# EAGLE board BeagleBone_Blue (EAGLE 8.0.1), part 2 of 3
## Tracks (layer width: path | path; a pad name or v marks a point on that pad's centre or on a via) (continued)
GND  (via drill 0.25 pad 0.46, 0.41, 0.5) (continued)
  Top 0.406: H2.3 79.3,24.38 | H2.4 79.96,24.41 | 83.84,22.52 83.84,24.43 | H2.9 83.21,24.43 | H2.18 81.92,27.46 | H1.9 74.65,16.76 | H1.10 74.65,17.41 74.65,17.4 | H1.3 74.62,12.86 74.62,12.85 | H1.4 74.62,13.51 | 74.62,13.51 | C38.2 46.13,45.99 v46.13,44.83 | C3.2 v49.15,42.88 | D9.A v60.45,53.39 | H1.18 71.6,15.46 71.6,15.47 | 5VREG.4 52.32,46.6 52.58,46.86 v52.58,47.62 | C5.2 50.64,43.3 v50.22,42.88 | R64.1 R63.1 R62.1 R61.1 R21.2 R22.2 20.75,2.23 v20.5,2.49
  Bottom 0.152: U13.H10 30.62,34.44 v31.62,34.44 | v31.62,34.44 32.62,34.44 U13.G5 33.12,34.69 v33.38,34.95 v33.37,34.95 U13.C4 | U13.K8 31.62,33.44 v31.62,34.44 | U13.E7 31.62,35.44 v31.62,34.44 | U13.N5 U13.P6 32.36,31.19 32.72,30.84 33.02,30.84 U13.P4 33.73,30.84 34.04,30.84 34.37,31.17 U13.N2 34.37,31.21 34.39,31.19 34.39,31.17 34.72,30.84 35.03,30.84 35.89,31.7 v35.89,32.51 | X2.6 3.36,31.03 v3.38,31.01 | X2.GND 15.76,28.79 15.93,28.96 v16.84,28.96 | 56.03,40.66 R143.1 56.03,40.56 56.16,40.44 v56.57,40.44 | R16.1 v65.15,37.85 | R17.1 v65.15,36.7 | R129.1 64.95,35.56 65.15,35.76 v65.15,36.04 | R135.1 v65.15,34.42 | R115.1 v65.15,30.99 | R131.1 v65.15,32.13 | R113.1 v65.18,29.84 | R25.2 v69.22,10.92 | R110.2 56.39,14.45 56.54,14.6 v56.97,14.6 | R14.2 58.73,14.45 58.88,14.6 v59.31,14.6 | v58.22,20.37 58.22,19.91 58.4,19.74 R158.2 | C27.2 v32.21,6.93 | C40.2 v48.9,9.55 | R59.1 49.35,10.77 49.25,10.87 49.25,11.02 49.15,11.12 v48.69,11.12 | v60.27,17.53 60.27,18.41 C41.2
  Bottom 0.254: C23.1 v67.74,22.02 | TP12.TP v69.39,2.64 | C2.1 v76.2,19.89 | C25.2 v29.59,52.83 | C26.2 v31.11,52.83 | C20.1 52.06,52.44 52.32,52.7 52.32,53.01 v52.7,53.39 | R48.1 C21.1 53.8,51 R46.1 53.77,51.49 53.85,51.56 53.85,53.37 v53.87,53.39 | U4.4 5.53,9.52 C55.2 6.15,9.58 v6.48,9.91 | C34.1 v14.43,16.38 | v19.33,37.72 19.33,39.29 C52.2 | U9.TP 21.84,38.25 22.43,38.84 23.55,38.84 v24.13,38.25 | U9.11 22.6,37.8 22.91,37.8 23.19,38.08 v23.19,38.23 | R108.2 R89.2 22.84,27.18 v21.77,26.11 | C51.1 22.81,30.73 v23.24,31.17 | C49.1 v41.66,38.86 | C16.2 v49.81,8.2 | R150.2 v36.8,32.51 | R24.2 13.97,43.94 13.44,44.48 v11.58,44.48 | R47.1 55.24,46.53 55.4,46.38 55.4,46.05 55.5,45.95 v55.5,45.49 | C24.1 55.96,47.62 56.87,48.54 v58.22,48.54 | U5.2 v21.18,19.63 | C62.2 v17.63,7.14 | C28.2 v21.01,18.41 | C45.2 v16.28,9.45 | C61.1 20.45,14.07 v20.75,14.38 | C63.2 v24.69,12.09 | C33.2 22.89,14.63 v23.67,14.63 | U1.2 v36.2,11.05 | C46.2 17.87,15.08 18.16,15.37 v18.54,15.37
  Bottom 0.406: L4.1 v15.11,6.86 | X4.GND 5.13,39.65 5.38,39.9 5.38,43 v3.58,44.81 | D1.A 51.42,43.31 50.65,43.31 v50.22,42.88
  Bottom 0.813: R107.1 14.82,44.23 14.1,44.96 14.1,45.95 13.54,46.51 5.23,46.51 4.47,47.27 12V.OUT
  other vias: 6.22,25.78 6.22,27.05 6.22,28.32 6.22,29.59 6.22,30.86 6.22,32.13 6.22,33.4 6.22,34.67 6.22,35.94 7.49,35.94 8.76,35.94 12.57,35.94 11.3,33.4 11.3,34.67 11.3,30.86 10.03,30.86 8.76,30.86 7.49,30.86 7.49,25.78 8.76,25.78 10.03,25.78 11.3,25.78 11.3,27.05 11.3,28.32 11.3,29.59 12.57,30.86 13.84,30.86 16.38,33.4 16.38,32.13 16.38,28.32 16.38,27.05 16.38,25.78 15.11,25.78 13.84,25.78 12.57,25.78 16.38,35.94 15.11,35.94 18.16,51.94 18.16,52.83 19.05,51.94 20.83,52.83 19.05,52.83 19.94,52.83 19.94,51.94 20.83,51.94 37.47,52.96 36.45,52.96 35.43,52.96 34.42,52.96 33.4,52.96 37.47,50.42 36.45,50.42 35.43,50.42 33.4,50.42 34.42,50.42 13.84,35.94 16.38,34.67 10.03,35.94 11.3,35.94 15.11,30.86 16.38,30.86 16.38,29.59 4.06,26.67 3.17,26.67 2.29,26.67 5.08,23.88 5.08,22.99 5.08,22.1 4.32,20.83 3.56,20.83 4.32,20.07 3.56,20.07 2.79,22.1 2.79,22.99 2.79,23.88 2.79,24.77 2.79,25.65 6.58,42.04 6.58,41.22 6.48,40.41 6.1,39.57 6.58,42.85 40.36,23.75 40.36,40.56 41.63,40.56 42.95,40.56 50.6,40.67 51.77,40.67 61.65,40.39 62.33,40.39 50.5,26.42 51.79,25.17 53.09,27.48 54.33,26.42 53.06,26.44 51.79,26.42 51.82,27.51 50.52,27.69 48.13,30.38 50.52,28.57 54.33,25.15 49.28,29.16 53.06,25.15 49.23,40.67 48.01,40.67 40.34,22.68 54.36,32.51 55.63,26.11 54.36,27.38 50.55,25.17 20.7,5.21 20.7,5.97
  pour Route15 (rank 6): -1.27,55.88 87.63,55.88 87.63,-1.27 -1.27,-1.27
  pour Top (no thermals): 21.21,49.66 21.21,52.96 26.42,52.96 26.42,49.91 31.5,49.91 31.5,53.47 17.53,53.47 17.53,50.29 19.94,50.29 19.94,49.66
  pour Bottom (no thermals): 38.23,53.47 32.77,53.47 32.77,49.91 38.23,49.91
  pour Top (no thermals): 38.61,53.47 32,53.47 32,49.91 38.61,49.91
  pour Top (rank 4): 1.52,43.69 21.21,43.69 21.21,20.19 16.26,20.19 16.26,17.91 1.52,17.91
  pour Top: 75.18,10.8 75.18,21.84 77.22,21.84 77.22,24 84.84,24 84.84,27.81 76.2,27.81 76.2,29.59 73.66,29.59 73.66,25.27 73.03,25.27 73.03,20.32 71.12,20.32 71.12,10.8
  pour Bottom: 17.78,53.34 21.21,53.34 21.21,51.56 17.78,51.56
  pour Top (rank 3): 39.75,20.7 39.75,41.02 62.61,41.02 62.61,39.75 42.29,39.75 42.29,37.21 41.02,37.21 41.02,20.7
  pour Top: 47.37,32.13 47.37,30.86 49.91,28.32 49.91,24.51 52.45,24.51 53.72,23.24 54.99,23.24 54.99,24.51 56.26,25.78 57.53,25.78 57.53,30.86 54.99,33.4 53.72,33.4 52.45,32.13 51.18,32.13 49.91,30.86 48.64,32.13
  pour Bottom (rank 3, no thermals): 20.45,9.52 20.45,4.83 20.95,4.83 20.95,9.52
GNDA_ADC  (via drill 0.25 pad 0.46)
  Top 0.152: 53.8,16.89 SIP.A9 53.72,17.32 54.23,17.83 54.23,18.09 54.81,18.67 54.81,18.92 54.51,19.23 54.51,19.69 54.69,19.86 54.69,20.32 54.51,20.5 54.51,21.03 v54.81,21.34 54.99,21.51 SIP.E8 | SIP.A6 57.53,16.59 v57.23,16.28
  Bottom 0.152: v57.23,16.28 56.52,16.99 56.52,17.93 56.67,18.09 56.87,18.09 57.07,18.29 C42.2 C43.2 C44.2 57.07,21.34 56.92,21.49 54.97,21.49 v54.81,21.34
GPIO1_17  (via drill 0.25 pad 0.46)
  Top 0.152: GP0.4 45.18,6.59 45.62,6.15 v45.97,6.15 | SIP.V14 48.16,37.69 48.16,37.01 48.36,36.8 v48.36,36.58 | v65.46,16.92 64.95,16.41 63.68,16.41 63.4,16.69 63.4,17.14 62.99,17.55 v62.26,17.55
  Bottom 0.152: v65.46,16.92 65.46,20.37 64.75,21.08 64.75,22.5 55.88,31.37 53.16,31.37 51.46,33.07 51.46,33.63 51.13,33.96 50.09,33.96 49.45,34.59 49.45,35.48 v48.36,36.58 | v62.26,17.55 62.48,17.32 62.48,6.68 61.77,5.97 46.15,5.97 v45.97,6.15
GPIO1_25  (via drill 0.25 pad 0.46)
  Top 0.152: GP0.3 46.23,8.84 46.23,7.95 46.56,7.62 v46.56,6.48 | SIP.U16 44.83,36.8 v45.06,36.58
  Bottom 0.152: v46.56,6.48 46.76,6.27 61.65,6.27 62.18,6.81 62.18,16.18 61.77,16.59 61.77,21.54 54.71,28.6 52.05,28.6 49.78,30.86 49.53,30.86 48.23,32.16 48.23,32.36 47.57,33.02 47.3,33.02 46.66,33.66 46.66,34.39 46.23,34.82 46.23,35.51 45.64,36.09 45.36,36.09 45.06,36.4 v45.06,36.58
GPIO3_1  (via drill 0.25 pad 0.46)
  Top 0.152: SIP.H17 43.56,25.25 43.81,24.99 46.3,24.99 46.74,24.56 v46.74,24.21 | GP1.4 v35.03,6.15 | v35.15,18.49 35.15,17.35 34.24,16.43 33.53,16.43 v33.35,16.61
  Bottom 0.152: v46.74,24.21 46.74,24.03 46.35,23.65 45.09,23.65 44.83,23.39 44.12,23.39 41.71,20.98 40.59,20.98 38.43,18.82 35.48,18.82 v35.15,18.49 | v35.03,6.15 34.85,5.97 31.9,5.97 31.19,6.68 27.13,6.68 26.06,7.75 26.06,15.57 27.28,16.79 33.17,16.79 v33.35,16.61
GPIO3_2  (via drill 0.25 pad 0.46)
  Top 0.152: SIP.J15 46.48,27.05 47.27,26.26 47.57,26.26 47.85,25.98 47.85,24.08 v47.65,23.88 | GP1.3 36.04,4.59 v36.04,6.63 | v35.81,18.34 35.81,17.3 34.65,16.13 32.89,16.13 v32.72,16.31
  Bottom 0.152: v47.65,23.88 47.12,23.34 45.24,23.34 44.98,23.09 44.25,23.09 41.83,20.68 40.72,20.68 38.56,18.52 35.99,18.52 v35.81,18.34 | v36.04,6.63 34.77,6.63 34.42,6.27 32.05,6.27 31.34,6.98 27.25,6.98 26.36,7.87 26.36,15.44 27.41,16.48 32.54,16.48 v32.72,16.31
GPIO3_17  (via drill 0.25 pad 0.46)
  Top 0.152: SIP.C12 v50.55,18.8 | v46.13,11.25 44.15,11.25 43.18,10.29 GP0.6
  Bottom 0.152: v50.55,18.8 49.25,18.8 48.62,18.16 48.62,16.38 46.94,14.71 46.76,14.71 46,13.95 46,12.95 46.61,12.34 46.61,11.73 v46.13,11.25
GPIO3_20
  Top 0.152: GP0.5 44.18,9.91 44.78,10.52 46.13,10.52 46.61,11 46.61,12.14 47.04,12.57 47.65,12.57 48.67,13.59 48.67,14.4 49.43,15.16 49.43,18.14 48.69,18.87 48.41,18.87 48.16,19.13 48.16,19.66 48.64,20.14 SIP.D13
I2C0_SCL  (via drill 0.25 pad 0.46)
  Top 0.152: SIP.C16 44.83,19.1 44.73,19 v44.25,19 | SIP.C20 38.94,18.62 38.94,16.53 38.56,16.15 v38.15,16.15
  Bottom 0.152: R23.1 25.76,20.27 28.02,18.01 35.41,18.01 37.26,16.15 v38.15,16.15 38.41,16.15 41.25,19 v44.25,19
  Bottom 0.254: U5.1 22.99,20.57 23.29,20.27 R23.1
I2C0_SDA  (via drill 0.25 pad 0.46)
  Top 0.152: SIP.C17 43.56,18.8 43.71,18.64 43.89,18.64 v44.2,18.34 | SIP.C19 40.34,18.74 39.55,18.74 39.24,18.44 39.24,16.15 v38.76,15.67
  Bottom 0.152: R2.1 26.59,19 27.89,17.7 35.28,17.7 37.31,15.67 v38.76,15.67 38.76,16.08 41.02,18.34 v44.2,18.34
  Bottom 0.254: U5.3 22.96,18.69 23.27,19 R2.1
I2C1_SCL  (via drill 0.25 pad 0.46)
  Top 0.152: SIP.A16 44.83,16.36 44.96,16.23 v44.96,15.8 | v36.4,7.7 36.05,8.04 I2C.3
  Bottom 0.152: v44.96,15.8 44.78,15.62 40.69,15.62 39.65,14.58 34.04,14.58 32.74,13.28 32.74,9.73 33.71,8.76 35.33,8.76 v36.4,7.7 36.4,7.37 36.6,7.16 R12.1
I2C1_SDA  (via drill 0.25 pad 0.46)
  Top 0.152: v44.35,16.1 44.35,17.09 44.83,17.58 SIP.B16 | v35.71,7.7 35.28,7.7 35.05,7.92 I2C.4
  Bottom 0.152: v44.35,16.1 44.17,15.93 40.56,15.93 39.52,14.88 33.91,14.88 32.44,13.41 32.44,9.6 33.58,8.46 34.31,8.46 35.08,7.7 v35.71,7.7 35.71,7.31 35.56,7.16 R13.2
I2C2_SCL  (via drill 0.25 pad 0.46)
  Top 0.152: BMP.4 28.46,23.1 | BMP.4 28.21,23.05 27.96,23.29 R11.1 27.48,23.67 27.28,23.88 25.45,23.88 25.17,24.16 25.17,24.87 25.3,24.99 26.87,24.99 27.18,25.3 27.18,26.57 27.32,26.7 IMU.23 | BMP.4 28.46,22.72 28.93,22.25 32.69,22.25 33.12,21.82 35.69,21.82 37.19,20.32 v37.19,18.03 | SIP.D17 43.87,21.01 v43.87,21.36
  Bottom 0.152: v43.87,21.36 42.95,21.36 41.96,20.37 40.84,20.37 38.68,18.21 37.36,18.21 v37.19,18.03
I2C2_SDA  (via drill 0.25 pad 0.46)
  Top 0.152: BMP.3 29.11,23.11 | BMP.3 29.11,23.41 28.98,23.55 28.37,23.55 28.22,23.7 28.22,24.13 27.89,24.46 R10.2 27.48,25.83 27.71,26.06 IMU.24 | BMP.3 29.11,22.73 29.29,22.55 32.84,22.55 33.27,22.12 35.84,22.12 37.67,20.3 v37.67,17.58 | SIP.D18 42.29,20.4 v42.6,20.09
  Bottom 0.152: v37.67,17.58 38,17.91 38.81,17.91 40.97,20.07 42.57,20.07 v42.6,20.09
IMU_INT  (via drill 0.25 pad 0.46)
  Top 0.152: 31.16,28.3 IMU.12 31.84,28.3 32.23,27.91 32.23,24.51 32.51,24.23 32.51,23.34 33.43,22.43 35.97,22.43 38.15,20.24 v38.15,17.12 | SIP.A14 47.37,17.22 v46.76,17.83
  Bottom 0.152: v38.15,17.12 38.15,17.37 38.38,17.6 38.94,17.6 40.95,19.61 42.88,19.61 43.38,20.12 44.5,20.12 45.03,19.58 45.03,18.29 45.49,17.83 v46.76,17.83
L3
  Top 0.254: B2.C R33.1
L4
  Top 0.254: B3.C R32.1
LDO_PGOOD
  Top 0.152: SIP.B5 59.28,18.64 59.28,19.69 59.05,19.91 58.42,19.91 58.01,19.51 58.01,19.15 57.81,18.95 57.33,18.95 57.05,19.23 57.05,19.79 56.62,20.22 56.03,20.22 55.47,20.78 55.47,22.17 55.19,22.45 50.95,22.45 50.72,22.23 50.37,22.23 50.14,22.45 41.96,22.45 41.81,22.3 41.81,21.03 41.5,20.73 41.5,19.13 41.1,18.72 40.87,18.72 40.31,18.16 SIP.B20
LED_GRN  (via drill 0.25 pad 0.46)
  Top 0.152: SIP.T7 56.26,35.46 55.78,34.98 55.78,33.2 56.06,32.92 56.67,32.92 57.05,32.54 57.05,31.88 57.33,31.6 57.61,31.6 58.01,31.19 58.01,25.73 58.45,25.3 63.14,25.3 v63.22,25.38 | v24.66,5.46 22.61,5.46 22.35,5.71 G.A 22.35,7.42 22.63,7.7 31.09,7.7 31.73,7.06 31.73,5.03 32.18,4.57 GP1.6
  Bottom 0.152: v63.22,25.38 62.76,25.83 62.76,26.36 62.97,26.57 63.48,26.57 64.01,26.04 64.01,24.54 65.66,22.88 65.66,21.49 66.67,20.47 66.67,15.95 64.31,13.59 64.31,5.92 62.53,4.14 25.2,4.14 24.66,4.67 v24.66,5.46
LED_RED  (via drill 0.25 pad 0.46)
  Top 0.152: 56.26,34.7 SIP.R7 56.26,34.14 57.05,33.35 57.05,33.12 57.25,32.92 57.58,32.92 58.01,32.49 58.01,31.7 58.32,31.39 58.32,26.7 58.75,26.26 63.07,26.26 v63.25,26.09 | R.A 23.88,7.01 24.08,7.21 v24.64,7.21 27.76,7.21 27.94,7.39 30.96,7.39 31.42,6.93 31.42,4.14 32.03,3.53 33.81,3.53 34.02,3.74 GP1.5
  Bottom 0.152: v63.25,26.09 63.7,25.63 63.7,24.41 65.35,22.76 65.35,21.36 66.37,20.34 66.37,16.08 64.01,13.72 64.01,6.05 62.41,4.45 25.63,4.45 25.4,4.67 25.4,6.83 25.02,7.21 v24.64,7.21
MCASP0_ACLKR  (via drill 0.25 pad 0.46)
  Top 0.152: SIP.U18 41.66,36.58 v41.66,36.12 | 23.99,31.89 U10.20 23.99,31.99 24.18,32.18 25.32,32.18 25.93,32.79 26.95,32.79 27.36,33.2 27.36,34.04 27.51,34.19 v27.84,34.19
  Bottom 0.152: v41.66,36.12 41.17,36.12 40.28,35.23 40.28,32.08 39.5,31.29 35.92,31.29 35.15,30.53 32.54,30.53 28.88,34.19 v27.84,34.19
MCASP0_AXR0  (via drill 0.25 pad 0.46)
  Top 0.152: SIP.T16 44.07,35.18 v44.07,34.24 | U10.17 25.57,29.98 25.93,30.35 25.93,31.93 26.19,32.18 v27.84,32.18
  Bottom 0.152: v44.07,34.24 43.54,34.77 41.45,34.77 41.2,34.52 41.2,31.7 39.88,30.38 36.3,30.38 35.53,29.62 31.95,29.62 29.38,32.18 v27.84,32.18
MCASP0_AXR1  (via drill 0.25 pad 0.46)
  Top 0.152: SIP.V17 43.08,38 43.08,35.43 v43.26,35.25 | v27.84,33.5 28.19,33.5 28.32,33.38 28.32,31.88 28.14,31.7 27.58,31.7 27.41,31.88 26.39,31.88 26.24,31.72 26.24,30 25.73,29.49 U10.16
  Bottom 0.152: v43.26,35.25 42.72,35.79 42.22,35.79 41.96,35.53 41.02,35.53 40.59,35.1 40.59,31.95 39.62,30.99 36.04,30.99 35.28,30.23 32.34,30.23 28.89,33.68 28.02,33.68 v27.84,33.5
MCASP0_FSR  (via drill 0.25 pad 0.46)
  Top 0.152: SIP.V12 49.43,38.96 43.08,38.96 42.77,38.66 42.77,35.41 42.67,35.31 v42.47,35.31 | U10.18 25.51,30.48 25.63,30.61 25.63,32.05 26.06,32.49 27.1,32.49 27.46,32.84 v27.84,32.84
  Bottom 0.152: v42.47,35.31 42.39,35.23 41.15,35.23 40.89,34.98 40.89,31.83 39.75,30.68 36.17,30.68 35.41,29.92 32.14,29.92 29.38,32.69 27.99,32.69 v27.84,32.84
MDIR_1A  (via drill 0.25 pad 0.46)
  Top 0.152: H1.21 68.25,13.51 67.46,14.3 67.46,16.03 66.98,16.51 66.98,17.65 66.52,18.11 v64.67,18.11 | SIP.T13 49.4,35.18 49.4,34.47 49.68,34.19 50.14,34.19 50.55,33.78 v50.55,33.17
  Bottom 0.152: v64.67,18.11 64.85,18.29 64.85,20.07 64.14,20.78 64.14,22.23 55.6,30.76 52.91,30.76 50.55,33.12 v50.55,33.17
MDIR_1B  (via drill 0.25 pad 0.46)
  Top 0.152: H1.22 68.19,12.86 v67.79,13.26 | v61.7,15.98 62,15.98 62.36,15.62 64.59,15.62 v66.37,13.84 | SIP.U17 44.12,37.21 44.4,36.93 v44.4,36.55
  Bottom 0.152: v67.79,13.26 67.21,13.84 v66.37,13.84 | v61.7,15.98 61.47,16.2 61.47,21.41 54.59,28.3 51.92,28.3 49.66,30.56 49.4,30.56 47.93,32.03 47.93,32.23 47.45,32.72 47.17,32.72 46.35,33.53 46.35,34.27 45.92,34.7 45.92,35.38 45.52,35.79 45.03,35.79 44.4,36.42 v44.4,36.55
MDIR_2A  (via drill 0.25 pad 0.46)
  Top 0.152: H1.17 67.81,16.11 67.28,16.64 67.28,17.91 66.4,18.8 v62.87,18.8 | SIP.R13 48.08,34.11 v47.75,34.11
  Bottom 0.152: v62.87,18.8 62.87,21.74 55.09,29.52 52.43,29.52 50.16,31.77 49.91,31.77 49.15,32.54 49.15,32.74 47.78,34.11 v47.75,34.11
MDIR_2B  (via drill 0.25 pad 0.46)
  Top 0.152: SIP.V4 60.07,38.02 60.76,37.34 v60.76,36.73 | v67.89,16.76 H1.16 | v65.43,27.03 64.62,27.84 60.81,27.84 60.55,28.09 60.55,31.11 60.91,31.47 v62.33,31.47
  Bottom 0.152: v67.89,16.76 67.59,17.07 67.59,20.88 66.57,21.89 66.57,24.21 65.73,25.04 65.73,26.72 v65.43,27.03 | v60.76,36.73 61.06,36.42 61.32,36.42 61.49,36.25 61.49,35.92 61.77,35.64 62,35.64 62.41,35.23 62.41,34.75 62.66,34.49 62.66,34.14 62.97,33.83 63.17,33.83 63.32,33.68 R140.1 62.84,33.27 62.33,32.77 v62.33,31.47
MDIR_3A  (via drill 0.25 pad 0.46)
  Top 0.152: SIP.R4 60.53,34.67 v61.16,34.04 | H2.21 79.93,29.86 v79.93,30.94
  Bottom 0.152: 61.16,33.66 v61.16,34.04 61.16,30.94 62.79,29.31 62.79,28.85 62.94,28.7 R118.1 63.32,29.08 63.5,29.26 65.89,29.26 68.61,31.98 70.21,31.98 71.04,32.82 71.04,34.04 71.55,34.54 80.67,34.54 81.18,34.04 81.18,32.18 v79.93,30.94
MDIR_3B  (via drill 0.25 pad 0.46)
  Top 0.152: R116.1 65.96,44.7 65.66,44.4 65.66,40.23 v64.41,38.99 | SIP.R3 60.71,35.31 v60.55,35.31 | H2.22 79.31,30.98 78.87,31.42 77.72,31.42 76.17,32.97 76.17,33.96 75.21,34.92 74.19,34.92 73.51,35.61 73.51,40.03 v73.69,40.21
  Top 0.254: R77.1 R116.1
  Bottom 0.152: v60.55,35.31 60.55,35.81 59.97,36.4 59.97,37.06 61.57,38.66 62.48,38.66 63.02,39.19 63.5,39.19 63.7,38.99 v64.41,38.99 66.55,38.99 67.46,39.9 73.38,39.9 v73.69,40.21
MDIR_4A  (via drill 0.25 pad 0.46)
  Top 0.152: SIP.R1 63.09,33.88 62.28,33.88 v61.98,33.58 | H2.17 82.56,30.62 82.42,30.76 80.9,30.76 v80.72,30.94
  Bottom 0.152: v61.98,33.58 61.98,33.55 61.47,33.05 61.47,31.14 62.76,29.84 R113.2 63.32,30.2 63.52,30.4 66.57,30.4 68.45,32.28 70,32.28 70.71,33 70.71,34.21 71.42,34.92 80.9,34.92 81.48,34.34 81.48,31.7 v80.72,30.94
MDIR_4B  (via drill 0.25 pad 0.46)
  Top 0.152: SIP.R2 62.18,34.67 61.98,34.47 v61.98,34.27 | H2.16 83.21,30.66 82.8,31.06 82.45,31.06 v82.27,31.24
  Bottom 0.152: v61.98,34.27 62.48,33.76 62.48,33.38 61.77,32.66 61.77,31.27 62.05,30.99 R115.2 63.32,31.34 63.52,31.55 65.53,31.55 67.77,33.78 68.63,33.78 68.86,34.01 68.86,34.65 68.4,35.1 67.92,35.1 67.59,35.43 67.59,36.37 68.28,37.06 81.2,37.06 81.79,36.47 81.79,31.72 v82.27,31.24
MMC1_CLK
  Bottom 0.152: U13.M6 32.37,33.19 33.37,34.19 36.88,34.19 37.41,34.72 R66.1 R15.2
MMC1_CMD  (via drill 0.25 pad 0.46)
  Top 0.152: v28.57,39.09 R67.1 | SIP.V9 54.2,38.48 54.59,38.86 v54.59,39.22
  Bottom 0.152: U13.M5 32.38,31.7 31.86,31.7 29.36,34.2 29.36,38.28 28.57,39.06 v28.57,39.09 29.62,40.13 37.41,40.13 38.99,41.71 46.99,41.71 47.55,41.15 53.44,41.15 54.59,40 v54.59,39.22
MMC1_DAT0  (via drill 0.25 pad 0.46)
  Top 0.152: R68.1 34.29,38.86 v33.86,38.43 | SIP.U7 56.57,37.52 v56.9,37.52
  Bottom 0.152: U13.A3 33.86,37.71 v33.86,38.43 34.04,38.61 38.05,38.61 38.86,39.42 46.71,39.42 47.17,38.96 51.64,38.96 52.5,38.1 53.72,38.1 54,37.82 56.19,37.82 56.49,37.52 v56.9,37.52
MMC1_DAT1  (via drill 0.25 pad 0.46)
  Top 0.152: R69.1 v33.15,38.73 | SIP.V7 56.57,38.18 v56.9,38.18
  Bottom 0.152: U13.A4 33.37,38.51 v33.15,38.73 33.33,38.91 37.92,38.91 38.73,39.73 46.84,39.73 47.3,39.27 51.77,39.27 52.63,38.41 53.85,38.41 54.13,38.12 56.16,38.12 56.21,38.18 v56.9,38.18
MMC1_DAT2  (via drill 0.25 pad 0.46)
  Top 0.152: v32,39.04 R70.1 | SIP.R8 55.78,35.46 55.78,38.68 56.21,39.12 v56.44,39.12
  Bottom 0.152: v56.44,39.12 56.21,39.12 55.52,38.43 54.25,38.43 53.95,38.73 52.73,38.73 51.89,39.57 47.42,39.57 46.97,40.03 38.61,40.03 37.8,39.22 32.18,39.22 v32,39.04 32,38.56 U13.A5
MMC1_DAT3  (via drill 0.25 pad 0.46)
  Top 0.152: SIP.T8 54.76,36.17 v54.76,36.58 | R71.1 36.58,39.24 36.85,38.96 v36.85,37.64
  Bottom 0.152: U13.B2 34.89,36.68 35.85,37.64 v36.85,37.64 37.41,37.64 38.1,36.96 39.37,36.96 40.54,38.12 43,38.12 43.54,38.66 51.51,38.66 52.38,37.8 53.59,37.8 53.87,37.52 54.25,37.52 54.76,37.01 v54.76,36.58
MMC1_DAT4  (via drill 0.25 pad 0.46)
  Top 0.152: 54.99,37.24 SIP.U8 | 54.74,37.21 SIP.U8 | v54.1,36.58 54.1,36.73 54.59,37.21 SIP.U8 | R72.1 37.72,39.12 37.44,38.84 v37.44,38.12 37.44,37.39 37.21,37.16 v36.25,37.16
  Bottom 0.152: v54.1,36.58 54.1,36.86 53.47,37.49 52.25,37.49 51.38,38.35 43.66,38.35 43.13,37.82 40.69,37.82 39.52,36.65 37.85,36.65 37.34,37.16 v36.25,37.16 | U13.B3 34.81,38.12 v37.44,38.12
MMC1_DAT5  (via drill 0.25 pad 0.46)
  Top 0.152: R73.1 35.43,39.27 35.64,39.06 v35.64,34.92 | v53.09,36.93 53.09,37.34 53.47,37.72 54.81,37.72 54.99,37.9 SIP.V8
  Bottom 0.152: U13.B4 v35.64,34.93 v35.64,34.92 37.06,34.92 37.39,35.25 37.39,36.12 37.62,36.35 39.67,36.35 40.84,37.52 43.26,37.52 43.4,37.66 43.56,37.82 43.79,38.05 51.26,38.05 52.38,36.93 v53.09,36.93
MMC1_DAT6  (via drill 0.25 pad 0.46)
  Top 0.152: SIP.R9 53.21,34.67 52.73,35.15 51.94,35.15 51.66,35.43 51.66,38.89 51.99,39.22 v53.09,39.22 | R74.1 v30.86,39.04
  Bottom 0.152: U13.B5 32.37,37.69 31.39,37.69 30.86,38.23 v30.86,39.04 31.34,39.52 37.67,39.52 39.24,41.1 46.33,41.1 47.55,39.88 52.73,39.88 53.09,39.52 v53.09,39.22
MMC1_DAT7  (via drill 0.25 pad 0.46)
  Top 0.152: 53.75,35.94 SIP.T9 54.3,35.94 54.79,35.46 55.22,35.46 55.47,35.71 55.47,39.06 v55.63,39.22 | v29.72,39.06 R75.1
  Bottom 0.152: v55.63,39.22 55.14,38.73 54.38,38.73 53.95,39.17 53.95,39.73 53.49,40.18 47.7,40.18 46.48,41.4 39.12,41.4 37.54,39.83 30.48,39.83 v29.72,39.06 29.72,38.63 29.87,38.48 29.87,37.69 30.37,37.19 U13.B6
MMC2_CLK
  Bottom 0.152: R76.1 36.35,29.57 35.79,29.01 31.55,29.01 29.36,31.19 27.64,31.19 27.05,31.77 27.05,33.96 26.85,34.16 26.44,34.16 25.93,34.67 25.93,35.61 24.73,36.81 U9.13
MMC2_CMD  (via drill 0.25 pad 0.46)
  Top 0.152: SIP.J16 44.37,27.05 44.15,27.28 v44.15,27.69
  Route2 0.152: v44.15,27.69 43.36,28.47 41.05,28.47 39.01,30.5 31.55,30.5 28.96,33.1 28.96,34.59 28.57,34.98 27.23,34.98 26.9,34.65 v26.67,34.65
  Bottom 0.152: v26.67,34.65 26.39,34.65 26.24,34.8 26.24,35.74 24.67,37.31 U9.12
MMC2_DAT0  (via drill 0.25 pad 0.46)
  Top 0.152: SIP.J17 43.16,27.05 42.95,27.25 v42.95,27.69
  Route2 0.152: v42.95,27.69 42.47,28.17 40.92,28.17 38.89,30.2 31.42,30.2 28.65,32.97 28.65,34.42 28.4,34.67 27.48,34.67 27.36,34.54 27.36,33.96 26.98,33.58 v26.57,33.58
  Bottom 0.152: v26.57,33.58 25.63,34.52 25.63,35.48 24.8,36.31 U9.14
MMC2_DAT1  (via drill 0.25 pad 0.46)
  Top 0.152: SIP.J18 42.27,27.08 42.27,27.53 v42.11,27.69
  Bottom 0.152: v42.11,27.69 42.11,27.96 41.91,28.17 36.68,28.17 36.3,27.79 34.11,27.79 33.27,26.95 33.27,24.97 32.77,24.46 27.64,24.46 27.36,24.74 27.36,29.01 25.76,30.61 25.76,31.9 25.32,32.33 25.32,35.36 24.87,35.81 U9.15
MMC2_DAT2  (via drill 0.25 pad 0.46)
  Top 0.152: SIP.K15 45.52,28.32 45.24,28.04 v45.24,27.79 | v25.81,33.6 25.32,33.6 24.89,33.17 24.18,33.17 23.75,33.6 23.75,34.59 v24.46,35.31
  Bottom 0.152: v45.24,27.79 44.86,28.17 42.57,28.17 42.27,28.47 36.55,28.47 36.17,28.09 31.06,28.09 29.29,29.87 26.92,29.87 26.06,30.73 26.06,32.03 25.63,32.46 25.63,33.43 v25.81,33.6 | U9.16 v24.46,35.31
MMC2_DAT3  (via drill 0.25 pad 0.46)
  Top 0.152: SIP.H16 44.04,26.57 41.94,26.57 41.63,26.87 41.63,27.15 41.45,27.33 v41.45,27.69
  Bottom 0.152: U9.17 24.7,34.81 25.02,34.49 25.02,32.21 25.45,31.77 25.45,30.45 27.05,28.85 27.05,24.05 27.71,23.39 32.13,23.39 33.58,24.84 33.58,26.82 34.24,27.48 36.42,27.48 36.63,27.69 v41.45,27.69
MODE_BTN  (via drill 0.25 pad 0.46)
  Top 0.152: SIP.U6 57.53,36.8 56.74,36.02 56.74,34.21 57.07,33.88 57.86,33.88 58.01,33.73 58.01,32.97 58.32,32.66 58.32,31.83 58.8,31.34 59.05,31.34 59.28,31.11 59.28,27.08 59.79,26.57 64.26,26.57 v64.41,26.42 | v24.08,9.55 27.05,9.55 27.56,10.06 MOD.2
  Bottom 0.152: 64.54,26.42 v64.41,26.42 65.13,25.7 65.13,25.17 66.27,24.03 66.27,21.74 67.28,20.73 67.28,15.7 64.92,13.34 64.92,5.66 62.79,3.53 23.9,3.53 23.09,4.34 23.09,8.94 23.7,9.55 v24.08,9.55
MOT1A
  Top 0.152: H1.1 H1.2 76.2,12.04 76.2,11.94
  Top 0.813: M1.P$2 81.52,10.54 78.74,10.54 77.34,11.94 76.2,11.94 75.95,11.94
MOT1B
  Top 0.152: H1.6 H1.5 76.07,14.47 76.07,14.48
  Top 0.813: M1.P$1 82.66,14.46 81.92,13.72 81.92,12.95 80.64,11.68 79.25,11.68 77.72,13.21 77.72,14.1 77.34,14.48 76.07,14.48 75.95,14.48
MOT2A
  Top 0.152: H1.11 H1.12 76.24,18.71 75.95,18.41
  Top 0.813: M2.P$1 80.01,16.13 77.72,18.41 75.95,18.41
MOT2B
  Top 0.152: H1.8 H1.7 76.23,15.46 75.95,15.75
  Top 0.813: M2.P$2 79.36,12.97 78.74,13.59 78.74,14.86 77.85,15.75 75.95,15.75
MOT3A
  Top 0.152: H2.2 78.66,22.69 78.36,22.99 78.01,22.64 H2.1
  Top 0.813: M3.P$1 78.36,21.07 78.36,22.99
MOT3B
  Top 0.152: H2.6 H2.5 80.82,22.73 80.9,22.73
  Top 0.813: M3.P$2 80.66,17.92 81.41,18.67 81.41,20.32 80.9,20.83 80.9,22.73 80.9,22.99
MOT4A
  Top 0.152: H2.12 H2.11 84.6,22.61 84.84,22.61
  Top 0.813: M4.P$2 84.59,17.92 85.22,18.54 85.22,20.32 84.84,20.7 84.84,22.61 84.84,22.99
MOT4B
  Top 0.152: H2.7 H2.8 82.56,22.72 82.3,22.99
  Top 0.813: M4.P$1 82.3,21.07 82.3,22.99
MOT_STBY  (via drill 0.25 pad 0.46)
  Top 0.152: v67.94,14.81 H1.19 | v66.9,25.55 66.22,25.55 65.94,25.27 65.94,23.9 65.76,23.72 55.93,23.72 v55.63,23.42 | SIP.D14 47.93,20.7 48.46,21.23 v48.46,21.34 | H2.19 81.25,28.68 v80.85,28.27
  Bottom 0.152: v55.63,23.42 55.63,22.76 55.3,22.43 53.09,22.43 51.99,21.34 v48.46,21.34 | v80.85,28.27 80.85,28.83 80.42,29.26 76.33,29.26 76.1,29.03 76.1,27.61 75.34,26.85 71.91,26.85 71.09,26.04 67.64,26.04 67.16,25.55 v66.9,25.55 66.9,22 67.44,21.46 68.53,21.46 69.24,20.75 69.24,16.1 v67.94,14.81
N$1
  Top 0.254: R36.2 68.83,27.56 J2.P$1
N$2  (via drill 0.25 pad 0.46)
  Top 0.152: SIP.G17 43.89,24.18 v43.89,23.88
  Bottom 0.152: R57.1 6.93,34.75 6.78,34.59 6.78,34.24 6.58,34.04 5.71,34.04 5.08,33.4 3.17,33.4 2.66,32.89 X2.5 2.66,30.89 4.88,28.68 4.88,25.04 5.84,24.08 5.84,21.67 7.98,19.53 10.16,19.53 13.99,23.37 24.38,23.37 28.52,19.23 33.91,19.23 34.72,20.04 37.9,20.04 40.06,22.2 40.72,22.2 40.97,22.45 40.97,24.08 41.25,24.36 43.41,24.36 v43.89,23.88
N$3
  Top 0.152: R22.1 22.68,3.35 22.35,3.68 G.C
N$4  (via drill 0.25 pad 0.46)
  Top 0.254: v32.03,42.27 29.92,42.27 28.83,43.36 28.83,47.75 v29.11,48.03
  Bottom 0.254: BAL.2 29.54,47.35 C17.1 29.52,47.85 29.34,48.03 v29.11,48.03 | R30.2 42.04,43.16 41.91,43.03 38.41,43.03 36.88,41.5 32.11,41.5 C18.2 v32.03,42.27
N$5  (via drill 0.25 pad 0.46)
  Top 0.152: SIP.F17 43.1,23.24 v42.93,23.42
  Bottom 0.152: R26.1 3.28,16.36 4.06,17.14 X2.2 4.06,18.39 4.6,18.92 10.41,18.92 14.22,22.73 24.16,22.73 28.27,18.62 34.16,18.62 34.98,19.43 38.15,19.43 40.31,21.59 41.43,21.59 42.93,23.09 v42.93,23.42
  Bottom 0.254: R26.1 3.3,15.44
N$6
  Top 0.152: R21.1 24.64,3.4 24.64,4.45 24.5,4.58 R.C
N$7
  Top 0.254: R90.1 OSC1.1
N$8
  Bottom 0.254: R28.2 28.4,47.3 C17.2 28.4,46.91 28.91,46.41 BAL.1
N$9
  cutout Route2: 5.59,26.29 3.81,26.29 3.3,25.78 3.3,21.34 4.57,21.34 4.57,25.02 5.08,25.53 5.59,25.53
  cutout Route15: 5.59,26.29 3.81,26.29 3.3,25.78 3.3,21.34 4.57,21.34 4.57,25.02 5.08,25.53 5.59,25.53
N$10  (via drill 0.5)
  Top 0.254: v54.99,53.39 54.99,52.13 6VREG.7
  Bottom 0.254: C21.2 54.81,52.7 54.99,52.88 v54.99,53.39
N$11
  Bottom 0.254: 39.78,43.64 C15.2
  Bottom 0.406: R44.2 39.78,43.64 | PROT.5 35.01,43.02 35.61,43.61 C15.2
N$12  (via drill 0.25 pad 0.46)
  Top 0.152: SIP.D19 41.5,21.18 41.5,22.45 41.81,22.76 v50.55,22.76 55.32,22.76 55.78,22.3 55.78,21.39 55.93,21.23 56.59,21.23 56.74,21.08 56.74,20.52 57.53,19.74 SIP.C6
  Bottom 0.152: TP5.TP 49.99,22.76 v50.55,22.76
N$13
  cutout Route2: 5.59,36.2 4.95,36.2 4.57,36.58 4.57,40.39 3.3,40.39 3.3,36.2 4.06,35.43 5.59,35.43
  cutout Route15: 5.59,36.2 4.95,36.2 4.57,36.58 4.57,40.39 3.3,40.39 3.3,36.2 4.06,35.43 5.59,35.43
N$14
  Top 0.152: IMU.10 C6.1
N$15
  Top 0.254: CHGIC.15 21.61,50.95 22.05,51.38 C14.1
N$16  (via drill 0.5)
  Top 0.406: 5VREG.2 v49.02,45.44
  pour Bottom (no thermals): 44.32,48.51 50.42,48.51 50.42,47.62 52.07,47.62 52.07,46.1 49.66,46.1 49.66,45.09 48.51,45.09 48.51,46.1 44.32,46.1
N$17
  Top 0.254: CHG.C R3.2
N$18
  Top 0.254: R3.1 36.32,49.28 36.17,49.43 25.04,49.43 24.64,49.02 CHGIC.11
N$20
  Top 0.254: WIFI.C 21.89,22.73 R91.1
N$24
  Bottom 0.254: BAL.4 31.98,45.74 32.26,45.47 C19.1
N$25
  Top 0.254: R37.2 68.58,29.84 J2.P$2
N$26
  Top 0.254: SIP.M20 39.32,31.29 C30.1 37.01,31.29 36.58,30.86 R20.2 36.14,30.15 35.94,30.35 35.94,31.11 35.52,31.54 Y1.2
N$27
  Top 0.254: SIP.K20 39.32,27.89 C29.1 37.01,27.89 36.58,28.32 R20.1 36.14,29.03 35.94,28.83 35.94,27.94 35.64,27.64 Y1.1
N$28
  Bottom 0.152: U5.5 18.9,20.57 18.69,20.37 18.69,17.45 19,17.14 WP.P$1
  Bottom 0.254: R58.1 19.74,20.64 U5.5 19.62,20.6
N$29
  Bottom 0.254: BAL.7 29.54,42.37 29.29,42.11 28.73,42.11 28.52,41.91 C1.1 27.81,41.58 27.18,42.22 R34.2
N$30
  Top 0.254: R38.2 68.33,32.13 J2.P$3
N$31
  Top 0.254: SIP.L20 38.86,29.59 | 38.86,29.59 38.28,29.01 C29.2 | C30.2 38.28,30.18 38.86,29.59
N$32
  Top 0.254: SIP.H20 39.32,26.21 C31.1 37.01,26.21 36.58,25.78 R18.2 36.14,25.07 35.45,25.76 Y2.P$2
N$33
  Top 0.254: SIP.F20 39.32,22.81 C32.2 37.01,22.81 36.58,23.24 R18.1 36.14,23.95 35.45,23.26 Y2.P$1
N$34
  Top 0.254: SIP.G20 38.61,24.51 | 38.61,24.51 38.02,23.93 C32.1 | 38.61,24.51 38.02,25.09 C31.2
N$35  (via drill 0.25 pad 0.46)
  Top 0.152: SIP.B14 47.85,17.68 47.85,16.69 47.52,16.36 47.52,14.76 47.68,14.6 v47.68,14.2
  Bottom 0.152: EMU0.TP 47.75,14.12 v47.68,14.2
N$36  (via drill 0.25 pad 0.46)
  Top 0.152: SIP.C14 48.16,18.64 48.16,15.14 v48.01,14.99
  Bottom 0.152: EMU1.TP 46.86,14.2 47.65,14.99 v48.01,14.99
N$37  (via drill 0.25 pad 0.46)
  Top 0.152: SIP.A11 51.18,14.76 v50.98,14.55
  Bottom 0.152: v50.98,14.55 50.52,15.01 50.04,15.01 49.76,14.73 49.76,14.05 49.53,13.82 TDO.TP
N$38
  Top 0.254: R39.2 67.61,34.87 67.74,35 68.66,35 J2.P$4
N$39  (via drill 0.25 pad 0.46)
  Top 0.152: SIP.A12 49.91,14.96 v49.28,14.33
  Bottom 0.152: TCK.TP 48.64,13.69 v49.28,14.33
N$40  (via drill 0.25 pad 0.46)
  Top 0.152: SIP.B11 50.7,17.68 50.7,14.99 v50.24,14.53
  Bottom 0.152: v50.24,14.53 50.42,14.35 TDI.TP
N$41  (via drill 0.25 pad 0.46)
  Top 0.152: SIP.C11 51.66,18.95 v51.66,14.53
  Bottom 0.152: v51.66,14.53 51.31,14.17 TMS.TP
N$42  (via drill 0.25 pad 0.46)
  Top 0.152: SIP.B10 51.97,17.68 51.97,16.23 52.45,15.75 v52.45,14.53
  Bottom 0.152: v52.45,14.53 52.2,14.27 TRSTN.TP 52.2,11.28 51.69,10.77 R59.2
N$43
  Top 0.152: U7.57 18.16,30.86 18.29,30.99 R100.2
N$45  (via drill 0.25 pad 0.46)
  Top 0.152: SIP.L15 45.62,29.11 44.63,29.11 44.37,29.36 44.02,29.36 43.76,29.11 43.36,29.11 43.08,29.39 43.08,30.1 42.93,30.25 v42.93,30.48
  Bottom 0.152: R76.2 40.69,29.57 40.89,29.77 42.22,29.77 v42.93,30.48
N$47
  Top 0.152: R61.2 25.63,4.35 0.C
N$48
  Top 0.254: B1.C R29.1
N$49
  Top 0.254: B0.C R31.1
N$50
  Bottom 0.254: BAL.3 30.2,46.46 30.68,46.94 R27.2
N$51
  Top 0.254: R40.2 68.33,36.7 68.96,37.34 68.96,37.85 J2.P$5
N$52
  Top 0.254: R41.2 68.33,38.99 68.96,39.62 68.96,40.39 J2.P$6
N$53  (via drill 0.25 pad 0.46)
  Top 0.254: 6VREG.2 55.02,45.74 v54.76,45.49
  Bottom 0.254: C22.1 53.77,46.1 53.92,45.95 54.3,45.95 v54.76,45.49
N$54
  Top 0.254: R42.2 68.07,41.27 69.72,42.93 J2.P$19
N$55  (via drill 0.25 pad 0.46, 0.5)
  Top 0.254: v22.73,52.83 22.86,52.83 23.16,52.53 C14.2
  Bottom 0.254: v22.73,52.83 21.84,51.94 21.84,51.31 21.59,51.05 18.8,51.05 18.16,50.42 18.16,49.53 v18.41,49.28
  other vias: 17.53,49.28
  pour Top (rank 2): 21.72,49.02 21.72,49.15 19.18,49.15 19.18,49.78 16.89,49.78 16.89,48.89 19.18,48.89 19.18,49.02
  pour Bottom (no thermals): 17.14,49.66 18.8,49.66 18.8,46.23 25.53,46.23 25.53,43.43 18.03,43.43 18.03,48.64 17.14,48.64
N$56
  Top 0.254: R43.2 68.1,43.56 68.45,43.92 68.45,44.14 69.01,44.7 69.39,44.7 69.72,45.03 J2.P$20
N$57
  Top 0.152: R62.2 26.67,4.33 1.C
N$58
  Top 0.152: R63.2 27.69,3.38 27.69,4.45 27.82,4.58 2.C
N$59
  Top 0.152: R64.2 29.64,3.35 29.97,3.68 3.C
N$60  (via drill 0.25 pad 0.46, 0.5)
  Bottom 0.254: v54.33,44.7 53.9,44.7 53.77,44.83 C22.2
  other vias: 62.1,47.75 63.12,47.75
  pour Bottom (no thermals): 60.33,48.64 63.75,48.64 63.75,47.12 65.66,47.12 65.66,44.45 57.53,44.45 57.53,47.12 60.33,47.12
  pour Top (no thermals): 53.34,47.24 54.23,47.24 54.23,45.09 58.93,45.09 58.93,48.64 63.75,48.64 63.75,46.86 59.82,46.86 59.82,44.45 53.34,44.45
N$61  (via drill 0.25 pad 0.46)
  Top 0.254: v56.16,45.49 57.33,45.49 57.56,45.72 6VREG.4
  Bottom 0.254: R47.2 55.98,46.15 56.16,45.97 v56.16,45.49
N$62  (via drill 0.25 pad 0.46, 0.5)
  Bottom 0.254: C23.2 67.74,25.25 68.17,25.68 71.65,25.68 v72.26,26.29
  Bottom 0.406: R49.2 56.9,50.42 57.12,50.19 58.04,50.19
  other vias: 71.75,51.18 72.77,51.18 72.77,52.07 71.75,52.07
  pour Top (no thermals): 71.37,25.78 73.15,25.78 73.15,52.7 71.37,52.7
  pour Bottom (no thermals): 73.28,52.7 57.53,52.7 57.53,50.04 73.28,50.04
N$63  (via drill 0.25 pad 0.46)
  Top 0.254: 6VREG.5 58.02,52.1 58.22,51.9 v58.22,49.23
  Bottom 0.254: R45.2 55.88,48.72 56.39,49.23 v58.22,49.23
N$65  (via drill 0.5)
  Top 0.254: v57.28,53.39 56.69,53.39 56.29,52.98 6VREG.6
  Bottom 0.254: R48.2 R49.1 56.9,53.01 v57.28,53.39
N$66
  Bottom 0.254: C24.2 R45.1
N$67  (via drill 0.25 pad 0.46)
  Top 0.254: CHGIC.10 v25.78,48.51
  pour Bottom (no thermals): 19.43,50.29 25.53,50.29 25.53,52.32 28.32,52.32 28.32,51.05 26.29,51.05 26.29,47.62 19.43,47.62
N$69
  Top 0.254: CHGIC.14 22.12,50.7 22.86,51.44 24.13,51.44 24.33,51.64 C10.2
N$70  (via drill 0.25 pad 0.46)
  Top 0.152: SIP.G15 45.64,24.51 v45.47,24.33
  Bottom 0.152: R54.1 9.22,33.58 8.87,33.22 8.2,33.22 6.48,31.5 5.97,31.5 5.2,32.27 X2.8 4.76,31.1 5.49,30.38 5.49,25.4 6.45,24.43 6.45,22.15 8.46,20.14 9.91,20.14 13.74,23.98 24.66,23.98 28.8,19.84 33.66,19.84 34.47,20.65 37.64,20.65 38.41,21.41 38.41,23.01 40.36,24.97 44.83,24.97 v45.47,24.33
N$71  (via drill 0.25)
  Top 0.152: R6.2 20.95,44.83 20.83,44.96 18.29,44.96 18.16,45.09 18.16,46.1 18.8,46.74 v19.25,46.74 | v23.24,50.8 22.99,50.8 22.63,50.44 CHGIC.13
  Top 0.254: R5.1 R6.2
  Bottom 0.152: v23.24,50.8 23.11,50.67 19.36,50.67 19.13,50.44 19.13,46.86 v19.25,46.74
N$74  (via drill 0.25 pad 0.46)
  Top 0.152: v41.45,23.88 41.45,24.18 41.78,24.51 SIP.G18
  Bottom 0.152: v41.45,23.88 41.45,22.5 40.84,21.89 40.18,21.89 38.02,19.74 34.85,19.74 34.04,18.92 28.4,18.92 24.26,23.06 14.12,23.06 10.29,19.23 4.17,19.23 3.36,18.42 X2.3 3.36,16.95 2.74,16.33 2.74,15.57 2.59,15.42 R56.1
N$75  (via drill 0.25 pad 0.46)
  Top 0.152: SIP.C15 46.1,18.97 v45.92,18.8
  Bottom 0.152: R65.1 17.88,17.83 18.87,16.84 23.7,16.84 24.43,16.1 25.73,16.1 27.03,17.4 35.15,17.4 37.36,15.19 39.4,15.19 41.1,16.89 45.64,16.89 46.35,16.18 47.12,16.18 47.7,16.76 47.7,18.01 47.09,18.62 46.1,18.62 v45.92,18.8
  Bottom 0.254: X2.CD 14.75,18.4 15.32,17.83 R65.1
N$77  (via drill 0.25 pad 0.46)
  Top 0.152: SIP.G16 44.83,23.98 44.73,23.88 v44.55,23.88
  Bottom 0.152: R55.1 7.34,33.3 6.81,32.77 5.59,32.77 5.33,33.02 4.32,33.02 4.06,32.76 X2.7 4.06,31.37 5.18,30.25 5.18,25.22 6.15,24.26 6.15,21.92 8.23,19.84 10.03,19.84 13.87,23.67 24.54,23.67 28.68,19.53 33.78,19.53 34.59,20.34 37.77,20.34 38.71,21.28 38.71,22.88 40.49,24.66 44.3,24.66 44.55,24.41 v44.55,23.88
N$79
  Top 0.406: C3.1 47.36,44.39 47.37,44.4 47.37,45.09 47.75,45.47 5VREG.1 47.25,46.6 46.86,46.99 46.86,47.37 46.6,47.64 D3.C
  Top 0.813: D2.C D3.C
N$81  (via drill 0.25 pad 0.46)
  Top 0.152: C36.1 37.54,34.8 v36.85,35.48
  Bottom 0.152: U13.C2 35.58,35.48 v36.85,35.48
N$85  (via drill 0.25 pad 0.46)
  Top 0.152: 53.72,37.24 SIP.U9 53.72,36.88 53.62,36.78 53.62,36.58 53.31,36.27 v53.09,36.27
  Bottom 0.152: R15.1 39.62,35.86 40.97,37.21 43.38,37.21 43.92,37.74 51.13,37.74 52.6,36.27 v53.09,36.27
N$86  (via drill 0.25 pad 0.46)
  Top 0.152: v61.98,36.12 61.67,36.42 61.14,36.42 60.96,36.25 60.53,36.25 60.07,36.7 SIP.U4
  Bottom 0.152: R135.2 63.32,34.82 63.17,34.98 62.94,34.98 62.71,35.2 62.71,35.38 v61.98,36.12
N$103
  Top 0.152: U7.14 7.83,37.62 8.33,38.12 8.84,38.12 10.03,39.32 R84.2 10.92,39.73 10.77,39.88 10.49,39.88 10.39,39.98 10.39,41.43 10.57,41.6 R9.2
N$104
  Top 0.152: U7.13 8.53,37.66 8.69,37.82 8.97,37.82 9.83,38.68 11.23,38.68 11.86,39.32 R83.2
N$105
  Top 0.152: U7.12 9.23,37.65 9.96,38.38 11.43,38.38 11.73,38.68 12.68,38.68 13.31,39.32 R82.2
N$106
  Top 0.152: U7.11 9.93,37.72 10.29,38.08 11.58,38.08 11.89,38.38 12.85,38.38 13.16,38.68 14.94,38.68 15.11,38.86 R81.2
N$107
  Top 0.152: U7.10 10.63,37.6 10.79,37.77 11.73,37.77 12.04,38.08 13.01,38.08 13.31,38.38 16.15,38.38 16.51,38.73 R80.2
N$108
  Top 0.152: U7.8 12.03,37.61 12.19,37.77 13.16,37.77 13.46,38.08 17.63,38.08 17.91,38.35 R78.2
N$110  (via drill 0.25 pad 0.46)
  Top 0.152: SIP.B9 53.72,18.54 53.98,18.8 v54.25,18.8
  Bottom 0.152: R111.2 C42.1 | C42.1 C43.1 | v54.25,18.8 54.79,18.8 54.91,18.67 C42.1
N$111
  Top 0.152: U7.6 13.43,37.61 13.59,37.77 18.69,37.77 19.3,38.38 R79.2
N$112
  Top 0.152: U7.50 18.18,25.96 18.36,25.78 R85.2
N$113
  Top 0.152: U7.51 18.18,26.66 18.34,26.82 R86.2
N$114
  Top 0.152: U7.52 18.11,27.36 18.26,27.51 18.26,27.71 18.41,27.86 R92.2
N$115  (via drill 0.25 pad 0.46)
  Top 0.152: SIP.C9 53.24,18.95 53.24,16.69 53.52,16.41 54,16.41 54.3,16.71 54.3,17.04 v54.79,17.53
  Bottom 0.152: R109.2 R110.1 55.98,15.16 55.35,15.8 55.35,16.31 55.14,16.51 55.14,17.17 v54.79,17.53
N$116
  Top 0.152: U7.53 18.08,28.06 18.26,28.25 18.26,28.73 18.44,28.91 R96.2
N$121  (via drill 0.25 pad 0.46)
  Top 0.152: SIP.P15 45.54,33.4 45.24,33.1 45.24,32.84 45.01,32.61 41.83,32.61 v41.68,32.46 | R149.1 8.74,41.6 v9.6,41.6
  Route2 0.152: v41.68,32.46 41.12,32.46 40.39,31.72 32.05,31.72 30.18,33.6 30.18,35.56 27.99,37.74 v27.79,37.74
  Bottom 0.152: v9.6,41.6 10.03,42.04 24.89,42.04 26.95,39.98 26.95,38.25 27.46,37.74 v27.79,37.74
N$126  (via drill 0.25 pad 0.46)
  Top 0.152: SIP.P17 44.02,33.4 v44.2,33.58
  Bottom 0.152: v44.2,33.58 44.2,33.66 44.55,34.01 44.55,34.98 44.07,35.46 43.74,35.46 42.6,36.6 41.22,36.6 39.98,35.36 39.98,32.89 39.6,32.51 R150.1
N$128
  Bottom 0.406: X3.4 11.79,6.86 13.59,6.86 15.11,8.38 L4.2
N$129  (via drill 0.25 pad 0.46)
  Top 0.152: SIP.T18 41.71,35.36 v41.71,34.29 | v30.33,21.08 29.77,21.64 24.84,21.64 23.52,20.32 23.52,17.02 23.14,16.64 19.76,16.64 19.33,16.2 v19.33,14.43
  Bottom 0.152: v41.71,34.29 41.71,33.93 42.55,33.1 43.13,33.1 44.53,31.7 44.53,31.09 45.14,30.48 45.36,30.48 47.37,28.47 47.37,26.92 46.41,25.96 36.91,25.96 32.82,21.87 31.11,21.87 v30.33,21.08 | R156.1 v19.33,14.43
N$130
  pour Bottom (no thermals): 16.89,14.48 16.89,13.59 13.08,13.59 11.43,12.06 10.72,11.43 9.98,11.43 9.42,11.99 9.42,12.98 9.96,13.51 11.02,13.51 12.19,14.48
N$131  (via drill 0.25 pad 0.46)
  Top 0.152: SIP.B4 59.74,17.83 v59.44,17.83
  Bottom 0.152: v59.44,17.83 59.05,18.21 R158.1
N$146
  Top 0.152: U7.56 18.15,30.16 18.36,29.95 R97.2
N$148
  Top 0.152: U7.58 18.12,31.56 18.26,31.7 18.26,31.9 18.39,32.03 R123.2
N$149
  Top 0.152: U7.60 18.2,32.96 18.31,33.07 R124.2
NTE  (via drill 0.25 pad 0.46)
  Top 0.152: SIP.F18 42.29,23.7 v42.11,23.88
  Bottom 0.152: v42.11,23.88 42.14,23.9 43.16,23.9 43.41,23.65 43.41,23.11 41.58,21.28 40.44,21.28 38.28,19.13 35.1,19.13 34.29,18.31 28.14,18.31 24.03,22.43 14.35,22.43 10.54,18.62 5,18.62 4.76,18.38 X2.1 4.76,16.95 4.32,16.51 R35.1
PAUSE_BTN  (via drill 0.25 pad 0.46)
  Top 0.152: SIP.T6 57.05,35.46 57.05,34.42 57.28,34.19 58.04,34.19 58.32,33.91 58.32,33.15 58.55,32.92 58.93,32.92 59.59,32.26 59.59,27.66 59.72,27.53 64.39,27.53 64.9,27.03 64.9,25.73 v64.64,25.48 | v24.08,8.84 24.49,9.25 27.3,9.25 30.15,12.09 PAU.2
  Bottom 0.152: v64.64,25.48 64.64,25.22 65.96,23.9 65.96,21.62 66.98,20.6 66.98,15.82 64.62,13.46 64.62,5.79 62.66,3.84 24.03,3.84 23.39,4.47 23.39,8.59 23.65,8.84 v24.08,8.84
PMIC_INT
  Top 0.152: SIP.B18 SIP.B19
PMIC_NWAKEUP  (via drill 0.25 pad 0.46)
  Top 0.152: SIP.C5 58.8,18.97 58.62,18.8 v58.34,18.8 | SIP.A19 41.48,16.89 41.66,16.71 v41.66,16.41
  Bottom 0.152: v58.34,18.8 57.71,19.43 57.71,22.55 56.36,23.9 55.37,23.9 55.14,23.67 55.14,22.94 54.94,22.73 52.96,22.73 51.87,21.64 49.23,21.64 48.74,22.12 46.02,22.12 45.64,21.74 45.64,19.89 46.61,18.92 47.22,18.92 48.01,18.14 48.01,16.64 47.24,15.88 46.23,15.88 45.52,16.59 41.83,16.59 v41.66,16.41
PMIC_PGOOD  (via drill 0.25 pad 0.46)
  Top 0.152: SIP.B15 45.62,17.68 45.62,16.69 45.92,16.38 v45.92,15.49 | SIP.A20 40.89,15.75 v40.89,15.14 40.89,14.33 39.32,12.75 U6.2
  Bottom 0.152: v45.92,15.49 45.74,15.32 41.07,15.32 v40.89,15.14
POWER_BTN  (via drill 0.25 pad 0.46)
  Top 0.152: POW.2 v17.4,15.6 | SIP.D20 38.63,19.58 38.63,16.81 38.46,16.64 36.78,16.64 36.2,17.22 36.2,17.88 36.37,18.06 36.37,18.87 36.12,19.13 35.1,19.13 33.96,17.98 v33.96,16.92
  Bottom 0.152: v17.4,15.6 18.34,16.53 23.57,16.53 24.31,15.8 25.86,15.8 27.15,17.09 33.78,17.09 v33.96,16.92
PRU_E_A  (via drill 0.25 pad 0.46)
  Top 0.152: SIP.V13 49.3,37.82 v49.3,36.96 | v79.78,41.66 80.05,41.39 E4.3
  Bottom 0.152: v49.3,36.96 49.81,36.96 50.06,36.7 50.06,34.85 50.34,34.57 56.62,34.57 61.85,39.8 65.08,39.8 67.77,42.49 78.94,42.49 v79.78,41.66
PRU_E_B  (via drill 0.25 pad 0.46)
  Top 0.152: SIP.U13 48.64,36.98 48.84,36.78 48.84,36.6 49.15,36.3 v49.35,36.3 | v79.65,40.97 80.24,40.39 E4.4
  Bottom 0.152: v49.35,36.3 49.58,36.3 49.76,36.12 49.76,34.72 50.22,34.27 56.74,34.27 61.98,39.5 65.2,39.5 67.89,42.19 78.44,42.19 v79.65,40.97
PWM_1A  (via drill 0.25 pad 0.46)
  Top 0.152: H1.23 68.03,12.21 67.16,13.08 67.16,15.9 66.67,16.38 66.67,17.09 66.27,17.5 v64.97,17.5 | SIP.U14 47.7,36.88 v47.7,36.58
  Bottom 0.152: v64.97,17.5 65.15,17.68 65.15,20.22 64.44,20.93 64.44,22.38 55.75,31.06 53.03,31.06 51.13,32.97 51.13,33.45 50.93,33.66 49.96,33.66 49.15,34.47 49.15,35.36 48.41,36.09 47.95,36.09 47.7,36.35 v47.7,36.58
PWM_1B  (via drill 0.25 pad 0.46)
  Top 0.152: H1.15 67.96,17.41 67.59,17.78 67.59,18.69 66.27,20.02 v64.21,20.02 | SIP.T14 48.01,35.31 v48.39,35.31
  Bottom 0.152: v64.21,20.02 63.83,20.4 63.83,22.1 55.47,30.45 52.78,30.45 50.55,32.69 50.29,32.69 50.06,32.92 50.06,33.12 48.84,34.34 48.84,35.13 48.67,35.31 v48.39,35.31
PWM_2A  (via drill 0.25 pad 0.46)
  Top 0.152: SIP.U10 51.97,36.73 51.97,35.71 52.22,35.46 52.93,35.46 53.24,35.15 53.95,35.15 54.2,34.9 54.2,34.47 53.92,34.19 53.57,34.19 53.09,33.71 v53.09,33.22 | v70.51,29.62 70.74,29.39 70.74,27.08 v70.23,26.57 | H2.23 78.64,29.85 v78.64,30.94
  Bottom 0.152: v53.09,33.22 53.09,32.46 53.57,31.98 56.13,31.98 60.3,27.81 66.7,27.81 68.5,29.62 v70.51,29.62 | v70.23,26.57 71.2,26.57 71.78,27.15 75.21,27.15 75.79,27.74 75.79,29.23 76.12,29.57 77.95,29.57 78.64,30.25 v78.64,30.94
PWM_2B  (via drill 0.25 pad 0.46)
  Top 0.152: SIP.T10 52.6,35.79 53.19,35.79 53.52,35.46 54.33,35.46 54.51,35.28 54.51,34.06 54.36,33.91 v54.36,33.22 | H2.15 83.86,30.8 83.39,31.27 83.08,31.27 82.83,31.52 v82.83,31.6 | v73.69,33 73.51,32.82 73.51,30.61 v73.99,30.12
  Bottom 0.152: v54.36,33.22 55.32,33.22 60.43,28.12 66.55,28.12 68.43,30 70.21,30 70.89,30.68 70.89,31.9 71.42,32.44 73.13,32.44 v73.69,33 | v73.99,30.12 74.24,29.87 77.52,29.87 78.16,30.5 78.16,31.14 78.44,31.42 78.87,31.42 79.12,31.17 79.12,30 79.38,29.74 82.35,29.74 82.83,30.23 v82.83,31.6
PWR_LED  (via drill 0.25 pad 0.46)
  Top 0.152: v10.57,44.45 10.57,44.98 10.85,45.26 12.32,45.26 12.57,45.52 ON.C
  Bottom 0.152: R24.1 11.46,43.56 v10.57,44.45
RESET  (via drill 0.25 pad 0.46)
  Top 0.152: SIP.A10 52.45,16.41 53.06,15.8 54.66,15.8 55.04,15.42 55.04,12.32 54.76,12.04 54.76,11.56 54.59,11.38 52.76,11.38 52.09,10.72 v52.09,10.29 | v41.81,8.38 41.81,9.02 40.95,9.88 40.95,11.53 40.39,12.09 38.26,12.09 U6.4 38.25,11.73 38.08,11.56 35.41,11.56 34.72,12.24 34.72,13.11 34.34,13.49 24.82,13.49 23.42,12.09 RST.2
  Top 0.254: RST.2 22.48,13.66 v21.01,15.14
  Bottom 0.152: v52.09,10.29 46.89,10.29 45.9,9.3 45.9,7.31 45.19,6.6 43.99,6.6 43.23,7.37 43.23,7.9 42.75,8.38 v41.81,8.38
  Bottom 0.254: C33.1 R60.1 21.23,15.67 21.01,15.44 v21.01,15.14
SD_BOOT
  Top 0.254: SD.2 68.83,50.16 67.61,48.95 R77.2
SERVO_EN  (via drill 0.25 pad 0.46)
  Top 0.152: 6VREG.8 53.09,52.1 v52.98,51.99 | v59.33,39.14 59.51,38.96 60.43,38.96 60.86,38.53 60.86,38.28 61.34,37.8 SIP.U3
  Bottom 0.152: v59.33,39.14 59.33,39.32 57.15,41.5 57.15,42.57 55.55,44.17 53.92,44.17 52.73,45.36 52.73,46.46 53.54,47.27 53.54,49.15 53.77,49.38 R46.2 53.24,49.86 52.98,50.11 v52.98,51.99
SPI1_MISO  (via drill 0.25 pad 0.46)
  Top 0.152: S1.2.4 v55.35,7.7 | SIP.B13 49.12,17.68 49.12,16.61 48.95,16.43 v48.95,15.88
  Top 0.254: S1.1.4 S1.2.4
  Bottom 0.152: v55.35,7.7 55.35,9.8 54.89,10.26 54.89,12.47 54.41,12.95 53.82,12.95 53.52,13.26 53.52,14.71 52.91,15.32 51.41,15.32 50.85,15.88 v48.95,15.88
SPI1_MOSI
  Top 0.152: SIP.D12 50.42,20.7 50.9,20.22 51.33,20.22 51.97,19.58 51.97,19.18 52.2,18.95 52.65,18.95 52.93,18.67 52.93,16.43 53.26,16.1 54.86,16.1 55.42,15.55 55.42,13.03 55.7,12.75 56.19,12.75 56.69,12.24 56.69,10.13 56.34,9.78 S1.2.3
  Top 0.254: S1.1.3 S1.2.3
SPI1_SCK  (via drill 0.25 pad 0.46)
  Top 0.152: SIP.A13 48.64,16.53 48.46,16.36 48.46,15.67 48.69,15.44 v48.69,15.11
  Top 0.254: S1.1.5 S1.2.5 v54.34,7.71 v54.33,7.7
  Bottom 0.152: v54.33,7.7 54.33,11.12 54.59,11.38 54.59,12.34 54.28,12.65 53.7,12.65 53.21,13.13 53.21,14.58 52.78,15.01 51.28,15.01 50.98,15.32 48.9,15.32 v48.69,15.11
SPI1_SS1  (via drill 0.25 pad 0.46)
  Top 0.152: S1.1.6 v53.34,6.76 | SIP.H18 42.77,26.26 43.87,26.26 44.17,25.96 44.17,25.65 44.53,25.3 46.53,25.3 46.69,25.15 v47.17,25.15
  Bottom 0.152: v53.34,6.76 53.52,6.58 61.52,6.58 61.87,6.93 61.87,14.35 60.86,15.37 60.86,21.16 57.51,24.51 47.8,24.51 v47.17,25.15
SPI1_SS2  (via drill 0.25 pad 0.46)
  Top 0.152: v53.34,7.7 S1.2.6 52.27,8.89 v52.17,8.99 | SIP.C18 42.77,18.95 42.77,15.01 42.6,14.83 42.6,12.37 42.72,12.24 42.72,9.96 42.6,9.83 42.6,7.98 42.93,7.64 v42.93,6.91
  Bottom 0.152: 53.34,8.43 v53.34,7.7 | v42.93,6.91 43.54,6.3 45.34,6.3 46.2,7.16 46.2,8.64 46.56,8.99 v52.17,8.99
SVO1  (via drill 0.25 pad 0.46)
  Top 0.152: SIP.U5 59.28,36.73 v59.28,35.31 | v61.98,28.6 62.18,28.8 64.29,28.8 65.53,27.56 R36.1
  Top 0.254: R36.1 R50.1
  Bottom 0.152: 59.28,35.03 v59.28,35.31 59.28,29.69 60.38,28.6 v61.98,28.6
SVO2  (via drill 0.25 pad 0.46)
  Top 0.152: SIP.V5 59.59,37.69 59.59,35.71 59.77,35.53 59.77,35.08 59.59,34.9 59.59,34.47 59.87,34.19 60.33,34.19 v60.48,34.04 | v61.98,29.29 62.15,29.11 64.31,29.11 64.49,29.29 65.66,29.29 65.94,29.01 65.94,28.8 66.04,28.7 R51.1
  Top 0.254: R37.1 R51.1
  Bottom 0.152: v61.98,29.29 61.98,29.64 60.48,31.14 v60.48,34.04 60.48,33.91
SVO3
  Top 0.152: R38.1 66.12,32.13 65.96,32.28 65.96,33.5 65.66,33.81 64.97,33.81 64.08,32.92 59.79,32.92 59.59,33.12 59.59,33.88 SIP.R5
  Top 0.254: R38.1 R52.1
SVO4
  Top 0.152: R53.1 66.5,32.87 66.65,32.72 66.93,32.72 67.06,32.59 67.06,30.58 66.9,30.43 66.04,30.43 65.63,30.84 65.63,32.41 65.43,32.61 59.66,32.61 59.28,33 59.28,33.68 58.78,34.19 58.6,34.19 58.12,34.67 SIP.R6
  Top 0.254: R39.1 R53.1
SVO5
  Top 0.152: SIP.T3 61.82,35.46 65.94,35.46 66.04,35.56 R125.2
  Top 0.254: R40.1 R125.2
SVO6
  Top 0.152: R127.2 66.5,37.47 66.7,37.26 66.9,37.26 67.06,37.11 67.06,35.18 66.88,35 65.91,35 65.76,35.15 61.39,35.15 60.6,35.94 SIP.T4
  Top 0.254: R41.1 R127.2
SVO7
  Top 0.152: SIP.T1 64.19,35.94 64.67,36.42 64.67,38.08 66.17,39.57 66.37,39.57 66.5,39.7 R120.1
  Top 0.254: R42.1 R120.1
SVO8
  Top 0.152: SIP.T2 63.12,36.45 64.01,36.45 64.36,36.8 64.36,38.2 65.96,39.8 65.96,42.29 66.09,42.42 R122.1
  Top 0.254: R43.1 R122.1
SYS_5V  (via drill 0.25 pad 0.46, 0.6)
  Top 0.254: v19,9.09 20.04,8.05 28.45,8.05 30.84,10.44 v33.43,10.44
  Route2 0.61: v81.41,16.28 82.42,17.3 82.42,30.07 83.8,31.45 83.8,32.16 83.49,32.46 v82.55,32.46
  Bottom 0.254: U8.3 19.37,9.09 v19,9.09 | v33.43,10.44 33.43,12.14 33.6,12.32 U1.3
  Bottom 0.61: v60.2,42.06 60.68,42.55 66.17,42.55 67.31,43.69 67.31,45.87 68.89,47.45 75.31,47.45 83.03,39.73 83.03,34.85 82.55,34.37 v82.55,32.46 | U8.3 19.68,8.65 19.68,4.57 22.02,2.23 67.51,2.23 73.23,7.95 76.61,7.95 81.41,12.75 v81.41,16.28
  Bottom 0.813: TP1.TP v60.2,42.06
  pour Top (rank 2): 59.46,39.42 59.46,42.75 60.73,42.75 60.73,39.4 60.4,39.12 59.74,39.12
  pour Bottom (rank 2, no thermals): 17.14,10.16 17.14,7.87 20.07,7.87 20.07,9.78 18.67,9.78 18.67,10.16
UART0_RX  (via drill 0.25 pad 0.46)
  Top 0.152: UT0.3 64.88,5.55 64.69,5.74 63.63,5.74 62.87,4.98 61.42,4.98 60.78,5.61 60.78,9.09 59.79,10.08 v59.41,10.08 | SIP.E15 46.61,21.97 47.09,21.49 v47.09,21.34
  Bottom 0.152: v47.09,21.34 47.57,20.85 51.1,20.85 54.3,17.65 54.3,17.17 54.84,16.64 54.84,15.77 55.91,14.71 55.91,13.64 56.74,12.8 59.94,12.8 60.5,12.24 60.5,10.92 59.66,10.08 v59.41,10.08
UART0_TX  (via drill 0.25 pad 0.46)
  Top 0.152: UT0.4 61.32,4.57 60.48,5.41 60.48,8.74 59.79,9.42 v59.41,9.42 | SIP.E16 45.47,21.34 v46.43,21.34
  Bottom 0.152: v46.43,21.34 46.43,20.98 46.86,20.55 50.98,20.55 54,17.53 54,16.99 54.53,16.46 54.53,15.65 55.6,14.58 55.6,13.51 56.62,12.5 59.82,12.5 60.2,12.12 60.2,11.07 59.69,10.57 59.05,10.57 58.88,10.39 58.88,9.7 59.16,9.42 v59.41,9.42
UART1_RX  (via drill 0.25 pad 0.46)
  Top 0.152: UT1.3 64.88,10.61 63.78,11.71 v59.41,11.71 | SIP.D16 45.62,19.91 v46.74,19.91
  Bottom 0.152: v59.41,11.71 56.54,11.71 54.99,13.26 54.99,14.33 53.92,15.39 53.92,16.13 53.39,16.66 53.39,17.25 50.7,19.94 48.54,19.94 48.18,19.58 47.62,19.58 47.3,19.91 v46.74,19.91
UART1_TX  (via drill 0.25 pad 0.46)
  Top 0.152: UT1.4 63.88,10.49 63.32,11.05 v59.41,11.05 | SIP.D15 46.74,20.7 46.91,20.52 46.91,20.42 47.12,20.22 47.73,20.22 v47.88,20.07
  Bottom 0.152: v59.41,11.05 59.66,11.05 59.89,11.28 59.89,11.99 59.69,12.19 56.49,12.19 55.3,13.39 55.3,14.45 54.23,15.52 54.23,16.28 53.7,16.81 53.7,17.4 50.85,20.24 48.06,20.24 v47.88,20.07
UART2_RX  (via drill 0.25 pad 0.46)
  Top 0.152: GPS.3 46.18,5.43 45.95,5.66 45.47,5.66 44.68,6.45 v44.68,7.7 | SIP.A17 43.56,15.19 43.74,15.01 v43.74,14.53
  Bottom 0.152: v43.74,14.53 43.74,14.17 44.98,12.93 44.98,8 v44.68,7.7
UART2_TX  (via drill 0.25 pad 0.46)
  Top 0.152: GPS.4 45.18,5.47 44.02,6.63 v44.02,7.7 | SIP.B17 43.56,17.6 44.04,17.12 44.04,16.64 43.87,16.46 43.87,15.37 44.4,14.83 v44.4,14.53
  Bottom 0.152: 44.4,14.25 v44.4,14.53 44.4,14.12 45.29,13.23 45.29,7.57 44.93,7.21 44.25,7.21 44.02,7.44 v44.02,7.7
UART3_CTSN  (via drill 0.25 pad 0.46)
  Top 0.152: U10.12 v24.97,26.92 | SIP.M17 44.04,31.34 v44.04,31.5
  Bottom 0.152: R89.1 23.95,27.18 24.21,26.92 v24.97,26.92 24.97,24.11 26.9,22.17 32.69,22.17 36.78,26.26 46.28,26.26 47.07,27.05 47.07,28.35 45.24,30.18 45.01,30.18 44.22,30.96 44.22,31.32 v44.04,31.5
UART3_RTSN  (via drill 0.25 pad 0.46)
  Top 0.152: U10.13 24.99,27.96 v25.81,27.96 | SIP.M18 42.62,30.86 v43.26,31.5
  Bottom 0.152: R108.1 23.95,28.52 24.16,28.32 24.59,28.32 24.95,27.96 25.79,27.96 v25.81,27.96 26.14,27.63 26.14,23.67 27.33,22.48 32.54,22.48 36.63,26.57 46.15,26.57 46.76,27.18 46.76,28.22 45.11,29.87 44.88,29.87 v43.26,31.5
UART3_RX  (via drill 0.25 pad 0.46)
  Top 0.152: U10.14 24.98,28.47 v26.24,28.47 | SIP.L17 43.81,29.84 v43.81,30.25
  Bottom 0.152: v26.24,28.47 26.44,28.27 26.44,23.8 27.46,22.78 32.38,22.78 36.47,26.87 46.02,26.87 46.46,27.3 46.46,28.09 44.98,29.57 44.76,29.57 44.07,30.25 v43.81,30.25
UART3_TX  (via drill 0.25 pad 0.46)
  Top 0.152: v25.81,28.98 v25.8,28.98 U10.15 | SIP.L16 45.31,30.07 46.33,30.07 46.58,29.82 46.58,27.86 46.41,27.69 v45.92,27.69
  Bottom 0.152: v25.81,28.98 26.49,28.98 26.75,28.73 26.75,23.93 27.58,23.09 32.26,23.09 33.88,24.71 33.88,26.7 34.37,27.18 45.41,27.18 v45.92,27.69
UART4_RX  (via drill 0.25 pad 0.46)
  Top 0.152: DSM2.P$3 74.19,4.75 70.46,4.75 68.99,6.22 68.99,7.7 68.07,8.61 68.07,10.41 66.9,11.58 66.9,12.47 65.81,13.56 65.81,13.97 64.47,15.32 v61.7,15.32 | SIP.T17 43.56,36.4 v43.74,36.58
  Bottom 0.152: v61.7,15.32 61.34,15.32 61.16,15.49 61.16,21.28 54.46,27.99 51.79,27.99 49.53,30.25 49.28,30.25 47.62,31.9 47.62,32.11 47.32,32.41 47.04,32.41 46.05,33.4 46.05,34.14 45.62,34.57 45.62,35.25 45.39,35.48 44.91,35.48 44.32,36.07 44.17,36.07 43.74,36.5 v43.74,36.58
